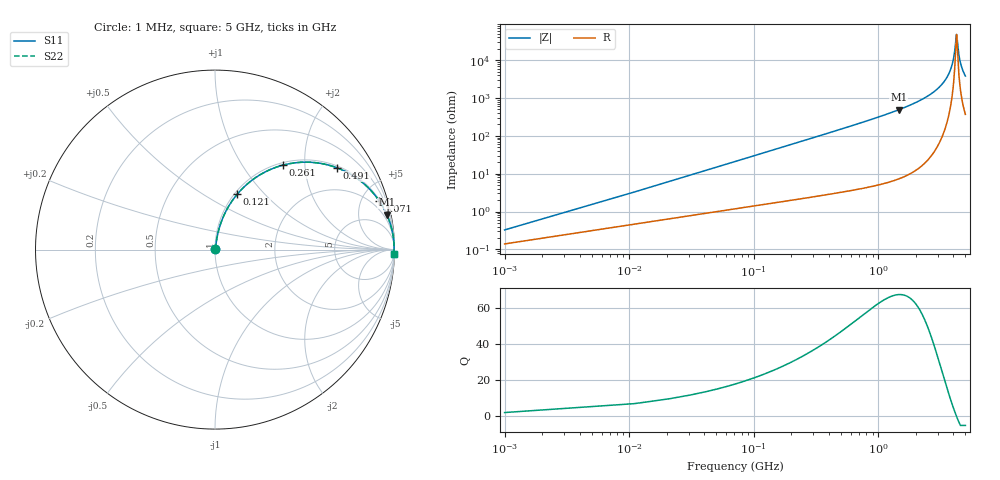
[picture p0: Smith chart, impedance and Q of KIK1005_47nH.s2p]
!version-3
!date-01.2023
!Series
# MHz S RI R 50
!Freq ReS11 ImS11 ReS21 ImS21 ReS12 ImS12 ReS22 ImS22
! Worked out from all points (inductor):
!   501 points, 1 MHz to 5 GHz, reference 50 ohm
!   read as one part in series: L = 47 nH near 21 MHz
!   highest Q = 67.2 at 1.461 GHz (marker M1), where L = 53.3 nH
!   self-resonance near 4.241 GHz
!   S11 on the Smith chart (normalised r, x): 1 MHz: 1.00, +0.01; 121 MHz: 1.03, +0.72; 261 MHz: 1.05, +1.55; 491 MHz: 1.06, +2.94; 1.071 GHz: 1.11, +6.76; 5 GHz: 8, -76
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1  0.0014 0.00294  0.9986 -0.00294  0.9986 -0.00294  0.0014 0.00294
31  0.0158 0.0894  0.9842 -0.0894  0.9842 -0.0894  0.0158 0.0894
41  0.0229 0.1173  0.9771 -0.1173  0.9771 -0.1173  0.0229 0.1173
71  0.0523 0.1964  0.9477 -0.1964  0.9477 -0.1964  0.0523 0.1964
121  0.1238 0.3086  0.8762 -0.3086  0.8762 -0.3086  0.1238 0.3086
261  0.3781 0.4705  0.6219 -0.4705  0.6219 -0.4705  0.3781 0.4705
491  0.68 0.4558  0.32 -0.4558  0.32 -0.4558  0.68 0.4558
841  0.8657 0.3326  0.1343 -0.3326  0.1343 -0.3326  0.8657 0.3326
1071  0.9159 0.2698  0.0841 -0.2698  0.0841 -0.2698  0.9159 0.2698
1461  0.9573 0.195  0.0427 -0.195  0.0427 -0.195  0.9573 0.195
1671  0.9692 0.1655  0.0308 -0.1655  0.0308 -0.1655  0.9692 0.1655
2501  0.9905 0.0874  0.00951 -0.0874  0.00951 -0.0874  0.9905 0.0874
3341  0.9968 0.0384  0.00324 -0.0384  0.00324 -0.0384  0.9968 0.0384
3891  0.9979 0.0139  0.00212 -0.0139  0.00212 -0.0139  0.9979 0.0139
4051  0.9979 0.00744  0.00205 -0.00744  0.00205 -0.00744  0.9979 0.00744
4171  0.9979 0.0028  0.00206 -0.0028  0.00206 -0.0028  0.9979 0.0028
4221  0.9979 0.000909  0.00208 -0.000909  0.00208 -0.000909  0.9979 0.000909
4251  0.9979 -0.000216  0.0021 0.000216  0.0021 0.000216  0.9979 -0.000216
4391  0.9978 -0.00536  0.0022 0.00536  0.0022 0.00536  0.9978 -0.00536
4521  0.9977 -0.01  0.00234 0.01  0.00234 0.01  0.9977 -0.01
4721  0.9973 -0.0169  0.00265 0.0169  0.00265 0.0169  0.9973 -0.0169
5000  0.9968 -0.0261  0.00323 0.0261  0.00323 0.0261  0.9968 -0.0261
